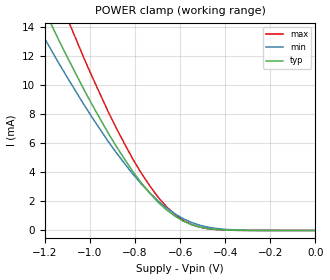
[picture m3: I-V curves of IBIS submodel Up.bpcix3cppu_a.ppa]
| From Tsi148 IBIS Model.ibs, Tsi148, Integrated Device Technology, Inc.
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[Submodel]  Up.bpcix3cppu_a.ppa
Submodel_type   Dynamic_clamp
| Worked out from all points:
|   POWER clamp passes 1 mA (typ) near -0.62 V on its own axis
[POWER Clamp]   | Note: Vtable = Vcc - Vout
| Voltage   I(typ)   I(min)   I(max)
-3.6V     104.9mA    87.57mA    127.3mA
-1.247V   16.68mA    14.5mA     20.41mA
-1.21V    15.46mA    13.49mA    18.93mA
-1.173V   14.27mA    12.49mA    17.46mA
-1.1V     11.95mA    10.55mA    14.62mA
-1.063V   10.82mA    9.607mA    13.24mA
-917mV    6.666mA    6.101mA    8.132mA
-807mV    4.01mA     3.839mA    4.852mA
-697mV    1.94mA     2.03mA     2.283mA
-623mV    987uA      1.15mA     1.106mA
-477mV    133uA      229uA      117uA
0V        0A         0A         0A
